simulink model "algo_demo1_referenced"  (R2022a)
settings: configuration reference "configurationSettings" (kept in a data dictionary, not in this file)
model workspace (MATLAB code in the model file):
  TP = algo_demo1_referenced_loadtp()
  TP = Simulink.Parameter(TP)
  TP.CoderInfo.StorageClass = 'Auto'
  FP = algo_demo1_referenced1_loadfp()

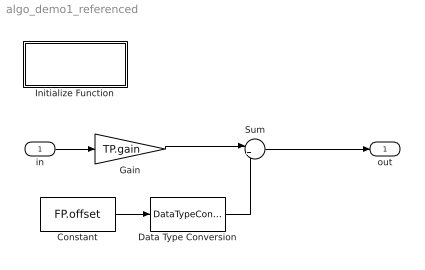
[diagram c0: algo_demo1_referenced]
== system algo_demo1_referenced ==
  in : Inport  OutDataTypeStr=single  Interpolate=off
  Constant : Constant  Value=FP.offset
  Data Type Conversion : DataTypeConversion  OutDataTypeStr=single
  Gain : Gain  Gain=TP.gain
  Initialize Function : Subsystem  TreatAsAtomicUnit=on
  Sum : Sum  Inputs=|++
  out : Outport  VectorParamsAs1DForOutWhenUnconnected=off
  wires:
  Gain/1 -> Sum/1
  in/1 -> Gain/1
  Sum/1 -> out/1
  Constant/1 -> Data Type Conversion/1
  Data Type Conversion/1 -> Sum/2

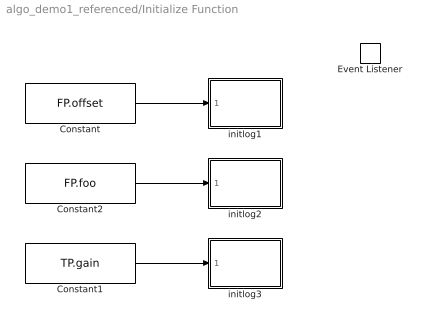
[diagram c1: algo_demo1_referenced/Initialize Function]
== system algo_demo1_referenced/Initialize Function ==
  Constant : Constant  Value=FP.offset
  Constant1 : Constant  Value=TP.gain
  Constant2 : Constant  Value=FP.foo
  Event Listener : EventListener  DisableCoverage=on  EventName=reset
  initlog1 : MATLAB Function  TreatAsAtomicUnit=on
  initlog2 : MATLAB Function  TreatAsAtomicUnit=on
  initlog3 : MATLAB Function  TreatAsAtomicUnit=on
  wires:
  Constant/1 -> initlog1/1(u)
  Constant1/1 -> initlog3/1(u)
  Constant2/1 -> initlog2/1(u)

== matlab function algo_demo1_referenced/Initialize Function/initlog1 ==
function fcn(u)

fprintf('refmodel fp.offset value is %f\n',u);

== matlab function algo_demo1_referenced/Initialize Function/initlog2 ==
function fcn(u)

fprintf('refmodel fp.foo value is %f\n',u);

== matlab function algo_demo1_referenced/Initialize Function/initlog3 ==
function fcn(u)

fprintf('refmodel tp.gain value is %f\n',u);
